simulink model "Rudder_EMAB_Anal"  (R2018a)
settings: Solver=ode45  StartTime=0.0  StopTime=1  RelTol=1e-3  EnableMultiTasking=on
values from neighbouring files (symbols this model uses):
  Be = 25    [init.m]
  Ja = 2.0e-4    (= 0.0002)    [init.m]
  Je = 2.2    [init.m]
  Jm = 5.0e-5    (= 5e-05)    [init.m]
  Kdmp = 0.001    [init.m]
  Keff = 0.85    [init.m]
  Kgs = 400.0    (= 400)    [init.m]
  Ki = 5.0    (= 5)    [init.m]
  Kl = 12/Kli    (= 1800000)    [init.m]
  Kmfr = 0.03    [init.m]
  Kp = 140    [init.m]
  Krfb = 0.0005    [init.m]
  Kt = 12/Kti    (= 1674418.60465)    [init.m]
  Kv = 260    [init.m]
  Ngear = 10.2    [init.m]
  Nscrew = 0.0026    [init.m]
  R = 0.287    [init.m]    (also in lqr_des.m = diag(R))
  Wmb = 1500    [init.m]

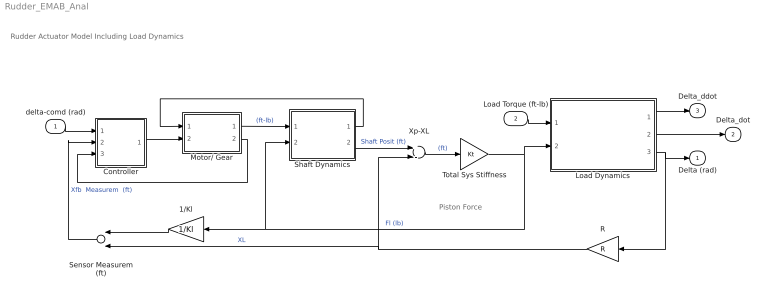
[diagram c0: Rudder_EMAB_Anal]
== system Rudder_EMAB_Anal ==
  note: Rudder Actuator Model Including Load Dynamics
  note: Piston Force
  delta-comd (rad) : Inport
  Load Torque (ft-lb) : Inport  Port=2
  1/Kl : Gain  Gain=1/Kl
  Controller : Subsystem
  Load Dynamics : Subsystem
  Motor/ Gear : Subsystem
  R : Gain  Gain=R
  Sensor Measurem (ft) : Sum
  Shaft Dynamics : Subsystem
  Total Sys Stiffness : Gain  Gain=Kt
  Xp-XL : Sum  Inputs=+-
  Delta (rad) : Outport
  Delta_dot : Outport  Port=2
  Delta_ddot : Outport  Port=3
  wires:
  Shaft Dynamics/2(Xp) -> Xp-XL/1  "Shaft Posit (ft)"
  Xp-XL/1 -> Total Sys Stiffness/1  "(ft)"
  Total Sys Stiffness/1 -> Load Dynamics/2(FL), 1/Kl/1, Shaft Dynamics/2(FL)  "Fl (lb)"
  Controller/1(V) -> Motor/ Gear/2(Vin)
  Motor/ Gear/1(Tm) -> Shaft Dynamics/1(Tq-mot)  "(ft-lb)"
  Load Dynamics/1(Del_ddot) -> Delta_ddot/1
  Load Dynamics/3(Delta (rad)) -> Delta (rad)/1, R/1
  Load Dynamics/2(Delta_dot) -> Delta_dot/1
  Sensor Measurem (ft)/1 -> Controller/2(Xp-fb)  "Xfb  Measurem  (ft)"
  Load Torque (ft-lb)/1 -> Load Dynamics/1(Load Torque)
  Shaft Dynamics/1(Xp-dot) -> Motor/ Gear/1(Xp-dot)
  R/1 -> Xp-XL/2, Sensor Measurem (ft)/2  "XL"
  Motor/ Gear/2(mr) -> Controller/3(rotor)
  delta-comd (rad)/1 -> Controller/1(delt-cmd)
  1/Kl/1 -> Sensor Measurem (ft)/1

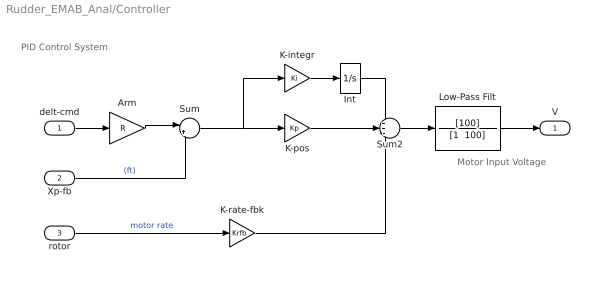
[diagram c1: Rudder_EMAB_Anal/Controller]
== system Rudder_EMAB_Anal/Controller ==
  note: PID Control System
  note: Motor Input Voltage
  delt-cmd : Inport
  Xp-fb : Inport  Port=2
  rotor : Inport  Port=3
  Arm : Gain  Gain=R
  Int : Integrator  UpperSaturationLimit=1  LowerSaturationLimit=-1
  K-integr : Gain  Gain=Ki
  K-pos : Gain  Gain=Kp
  K-rate-fbk : Gain  Gain=Krfb
  Low-Pass Filt : TransferFcn  Numerator=[100]  Denominator="[1  100]"
  Sum : Sum  Inputs=|+-
  Sum2 : Sum  Inputs=++-
  V : Outport
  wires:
  Arm/1 -> Sum/1
  K-rate-fbk/1 -> Sum2/3
  Int/1 -> Sum2/1
  K-integr/1 -> Int/1
  K-pos/1 -> Sum2/2
  Sum2/1 -> Low-Pass Filt/1
  rotor/1 -> K-rate-fbk/1  "motor rate"
  Xp-fb/1 -> Sum/2  "(ft)"
  delt-cmd/1 -> Arm/1
  Low-Pass Filt/1 -> V/1
  Sum/1 -> K-pos/1, K-integr/1

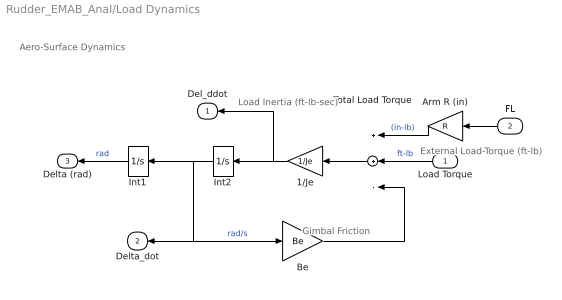
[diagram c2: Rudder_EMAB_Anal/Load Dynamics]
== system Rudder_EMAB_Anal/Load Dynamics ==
  note: Aero-Surface Dynamics
  note: Gimbal Friction
  note: Load Inertia (ft-lb-sec)
  note: External Load-Torque (ft-lb)
  Load Torque : Inport
  FL : Inport  Port=2
  1/Je : Gain  Gain=1/Je
  Arm R (in) : Gain  Gain=R
  Be : Gain  Gain=Be
  Int1 : Integrator
  Int2 : Integrator
  Total Load Torque : Sum  Inputs=++-
  Del_ddot : Outport
  Delta_dot : Outport  Port=2
  Delta (rad) : Outport  Port=3
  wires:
  Arm R (in)/1 -> Total Load Torque/1  "(in-lb)"
  Be/1 -> Total Load Torque/3
  Total Load Torque/1 -> 1/Je/1
  Int1/1 -> Delta (rad)/1  "rad"
  Load Torque/1 -> Total Load Torque/2  "ft-lb"
  FL/1 -> Arm R (in)/1
  Int2/1 -> Int1/1, Be/1, Delta_dot/1  "rad/s"
  1/Je/1 -> Int2/1, Del_ddot/1

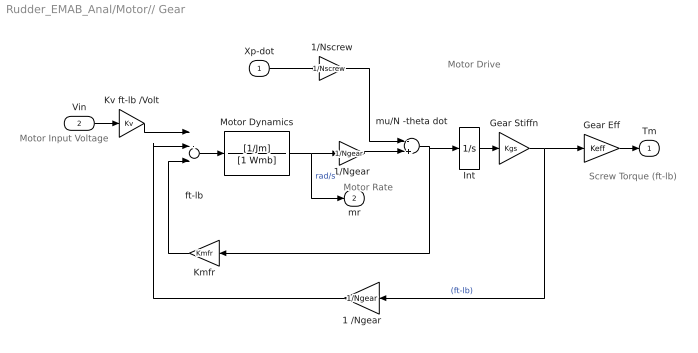
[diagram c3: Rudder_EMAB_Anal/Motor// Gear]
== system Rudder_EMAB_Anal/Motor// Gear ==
  note: Motor Drive
  note: Screw Torque (ft-lb)
  note: Motor Rate
  note: Motor Input Voltage
  Xp-dot : Inport
  Vin : Inport  Port=2
  1 /Ngear : Gain  Gain=1/Ngear
  1/Ngear : Gain  Gain=1/Ngear
  1/Nscrew : Gain  Gain=1/Nscrew
  Gear Eff : Gain  Gain=Keff
  Gear Stiffn : Gain  Gain=Kgs
  Int : Integrator  UpperSaturationLimit=0.4  LowerSaturationLimit=-0.4
  Kmfr : Gain  Gain=Kmfr
  Kv ft-lb /Volt : Gain  Gain=Kv
  Motor Dynamics : TransferFcn  Numerator=[1/Jm]  Denominator=[1 Wmb]
  ft-lb : Sum  Inputs=+---
  mu/N -theta dot : Sum  Inputs=-+
  Tm : Outport
  mr : Outport  Port=2
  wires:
  mu/N -theta dot/1 -> Int/1, Kmfr/1
  ft-lb/1 -> Motor Dynamics/1
  1 /Ngear/1 -> ft-lb/2
  Motor Dynamics/1 -> 1/Ngear/1, mr/1  "rad/s"
  1/Ngear/1 -> mu/N -theta dot/2
  Gear Stiffn/1 -> 1 /Ngear/1, Gear Eff/1  "(ft-lb)"
  Xp-dot/1 -> 1/Nscrew/1
  Vin/1 -> Kv ft-lb /Volt/1
  Gear Eff/1 -> Tm/1
  Kv ft-lb /Volt/1 -> ft-lb/1
  1/Nscrew/1 -> mu/N -theta dot/1
  Kmfr/1 -> ft-lb/3
  Int/1 -> Gear Stiffn/1

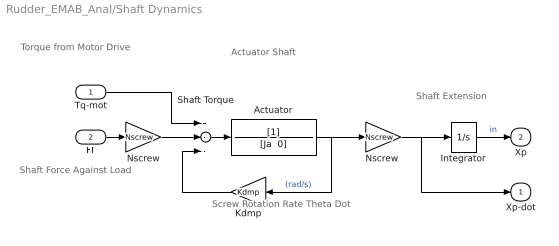
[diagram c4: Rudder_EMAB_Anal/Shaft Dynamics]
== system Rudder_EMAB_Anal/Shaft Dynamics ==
  note: Torque from Motor Drive
  note: Shaft Force Against Load
  note: Actuator Shaft
  note: Shaft Extension
  note: Screw Rotation Rate Theta Dot
  Tq-mot : Inport
  FL : Inport  Port=2
  Actuator : TransferFcn  Denominator="[Ja  0]"
  Integrator : Integrator
  Kdmp : Gain  Gain=Kdmp
  Nscrew : Gain  Gain=Nscrew
  "Nscrew " : Gain  Gain=Nscrew
  Shaft Torque : Sum  Inputs=+--
  Xp-dot : Outport
  Xp : Outport  Port=2
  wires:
  Actuator/1 -> "Nscrew "/1, Kdmp/1  "(rad/s)"
  Shaft Torque/1 -> Actuator/1
  Tq-mot/1 -> Shaft Torque/1
  Integrator/1 -> Xp/1  "in"
  FL/1 -> Nscrew/1
  Nscrew/1 -> Shaft Torque/2
  "Nscrew "/1 -> Integrator/1, Xp-dot/1
  Kdmp/1 -> Shaft Torque/3
